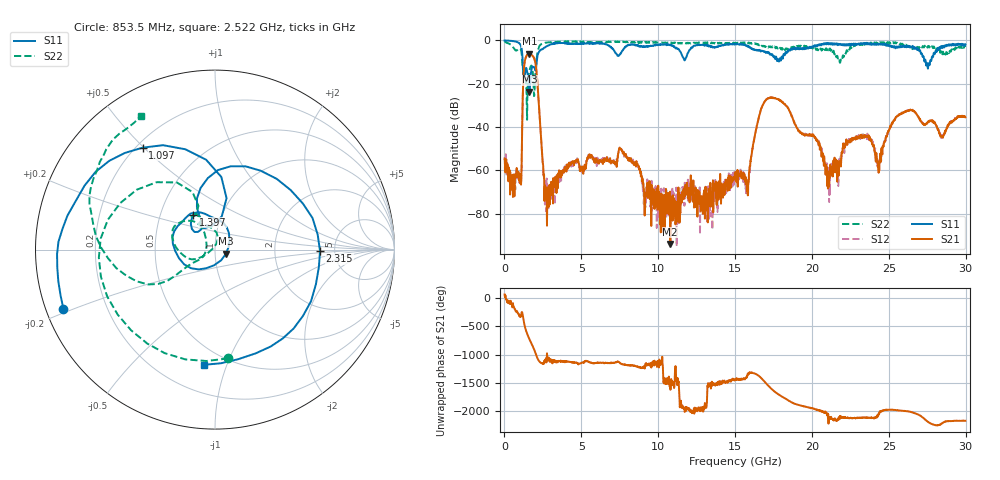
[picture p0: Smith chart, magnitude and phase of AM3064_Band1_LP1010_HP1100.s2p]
# Hz S DB R 50.0
!freq dBS11 angS11 dBS21 angS21 dBS12 angS12 dBS22 angS22
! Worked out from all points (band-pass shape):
!   1600 points, 10 MHz to 29.98 GHz, reference 50 ohm
!   highest |S21| = -6.12 dB at 1.622 GHz (marker M1); lowest = -94.1 dB at 10.79 GHz (marker M2)
!   |S21| within 3 dB of the highest: 1.338 GHz to 1.969 GHz (631.6 MHz wide, 38.2 % of centre)
!   lowest |S11| = -23.7 dB at 1.622 GHz (marker M3), VSWR 1.14, Z = 56.4 - j2.63 ohm
!   |S11| at or under -10 dB: 1.187 GHz to 2.096 GHz (909.2 MHz wide, 55.4 % of centre); 27.4 GHz to 27.68 GHz (280.5 MHz wide, 1.02 % of centre)
!   |S22| runs from -36.7 to -0.4 dB; largest |S21 - S12| = 0.0059
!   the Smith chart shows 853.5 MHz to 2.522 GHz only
!   S11 on the Smith chart (normalised r, x): 853.5 MHz: 0.05, -0.19; 1.097 GHz: 0.23, +0.50; 1.397 GHz: 0.73, +0.30; 2.315 GHz: 3.82, -0.09; 2.522 GHz: 0.38, -0.84
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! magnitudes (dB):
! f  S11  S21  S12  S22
! 10 MHz  0.0  -54.8  -53.8  -0.4
! 853.5 MHz  -0.8  -61.6  -64.3  -4.3
! 1.097 GHz  -3.1  -62.6  -65.2  -5.2
! 1.397 GHz  -12.8  -7.7  -7.7  -18.5
! 1.622 GHz  -23.7  -6.1  -6.1  -14.0
! 2.016 GHz  -13.9  -10.6  -10.5  -15.2
! 2.315 GHz  -4.7  -37.7  -37.9  -2.2
! 2.522 GHz  -3.8  -58.1  -60.8  -1.4
! 2.765 GHz  -2.6  -85.6  -69.9  -1.0
! 5.015 GHz  -1.4  -58.8  -60.7  -0.7
! 7.62 GHz  -5.3  -50.7  -50.4  -0.7
! 10 GHz  -2.0  -67.1  -81.4  -1.0
! 10.79 GHz  -2.3  -94.1  -75.7  -1.1
! 15 GHz  -1.8  -63.2  -64.6  -1.3
! 15.81 GHz  -2.9  -68.4  -65.7  -1.3
! 17.16 GHz  -5.5  -26.7  -26.6  -3.3
! 19.99 GHz  -3.4  -43.6  -44.0  -3.3
! 21.15 GHz  -1.4  -63.3  -71.2  -3.8
! 22.75 GHz  -2.3  -45.1  -45.7  -2.0
! 24.36 GHz  -1.8  -56.6  -57.0  -1.4
! 25 GHz  -2.0  -41.9  -41.7  -1.1
! 29.98 GHz  -1.8  -35.5  -35.1  -3.0
